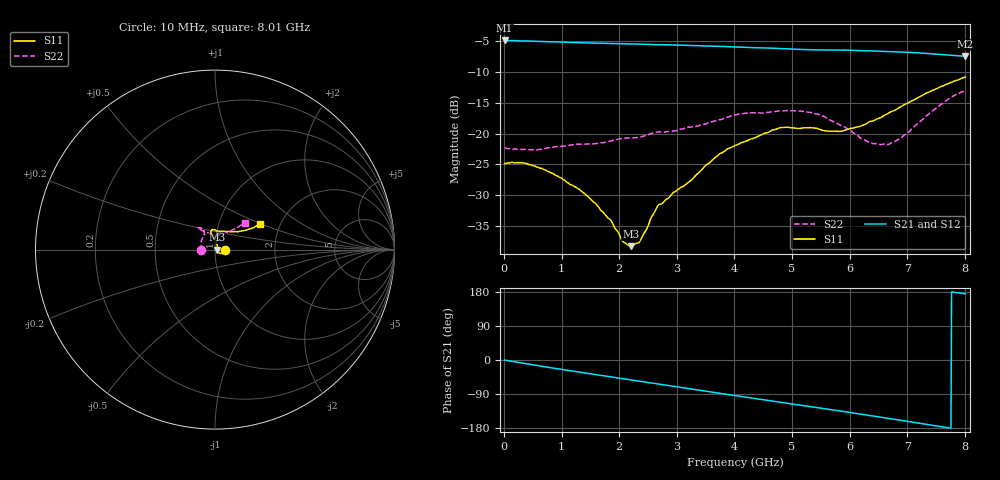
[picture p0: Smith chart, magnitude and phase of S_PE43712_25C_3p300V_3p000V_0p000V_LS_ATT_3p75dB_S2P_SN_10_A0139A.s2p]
! DEVICE ID: PE43712
! File Path: z:\PE43713\PE43713_CHAR_NOM_04292014\AMB\3p300\LS_ATT_3p75dB\PE43713_AMB_3p300V_3p000V_0p000V_LS_ATT_3p75dB_S2P_SN_10_A0139A.s2p
! Serial: 10
! Lot: A0139A
! Temp: 25C
! VDD: 3.300
! VSS: 0.000
! Control_Hi: 3.000
! Control_Lo: 0.000
! Attenuation Step: 3.75dB
! Port 1: RF1
! Port 2: RF2
! ThroughPath:1-2
! IDD: 0.0001469664
! ISS: -1.52e-007
#  Hz  S  RI  R  50
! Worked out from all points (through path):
!   801 points, 10 MHz to 8.01 GHz, reference 50 ohm
!   highest |S21| = -4.84 dB at 10 MHz (marker M1); lowest = -7.4 dB at 8.01 GHz (marker M2)
!   group delay of S21, straight-line fit = 63.6 ps
!   lowest |S11| = -38.3 dB at 2.2 GHz (marker M3), VSWR 1.02, Z = 51.2 - j0.0302 ohm
!   |S11| at or under -10 dB: start of sweep to end of sweep
!   |S22| runs from -22.7 to -13.1 dB; largest |S21 - S12| = 0.0017
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1e7  0.057 -0.00017  0.5726 -0.00318  0.5724 -0.00292  -0.0765 0.000338
3.4e8  0.0563 -0.0118  0.5605 -0.0876  0.5602 -0.0862  -0.0741 0.00417
6.3e8  0.0491 -0.018  0.5404 -0.1553  0.5402 -0.1553  -0.0738 0.00891
9.6e8  0.0388 -0.0212  0.5077 -0.2255  0.5077 -0.2255  -0.0769 0.0156
1.35e9  0.027 -0.0201  0.4602 -0.2981  0.4602 -0.2981  -0.0781 0.0248
1.6e9  0.021 -0.0162  0.425 -0.3402  0.4251 -0.34  -0.076 0.0332
1.85e9  0.0171 -0.01  0.3868 -0.3784  0.3868 -0.3782  -0.0755 0.0429
2.07e9  0.0123 -0.00446  0.3502 -0.4089  0.3502 -0.4087  -0.076 0.0507
2.2e9  0.0121 -0.000295  0.3274 -0.4255  0.3274 -0.4253  -0.0736 0.0554
2.36e9  0.0115 0.00667  0.2977 -0.4438  0.2977 -0.4436  -0.0692 0.0631
2.68e9  0.0139 0.0223  0.2373 -0.4727  0.2373 -0.4727  -0.0598 0.0842
3.22e9  0.00475 0.0403  0.1272 -0.5058  0.1273 -0.5058  -0.0602 0.0952
3.72e9  -0.00161 0.0669  0.0249 -0.5119  0.0247 -0.5118  -0.0653 0.111
4.01e9  -0.00968 0.0791  -0.0344 -0.5062  -0.0344 -0.5062  -0.0769 0.1191
4.79e9  -0.0201 0.1099  -0.1795 -0.4581  -0.1795 -0.4584  -0.0935 0.1212
5.35e9  -0.00593 0.1111  -0.2668 -0.401  -0.2667 -0.4007  -0.0922 0.1156
5.86e9  0.0248 0.1013  -0.3385 -0.3381  -0.338 -0.338  -0.0575 0.1005
6.32e9  0.0698 0.1008  -0.3895 -0.2658  -0.3886 -0.2656  -0.0171 0.0839
6.68e9  0.1081 0.0999  -0.4183 -0.2017  -0.4178 -0.2017  0.0171 0.0799
6.9e9  0.1325 0.1004  -0.4315 -0.1611  -0.431 -0.1611  0.0395 0.0838
7.71e9  0.2212 0.1267  -0.436 -0.00901  -0.4358 -0.00943  0.1377 0.1316
8.01e9  0.2506 0.1427  -0.4231 0.0389  -0.4223 0.0381  0.1651 0.149
